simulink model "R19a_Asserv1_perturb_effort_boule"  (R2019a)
settings: Solver=ode15s  StartTime=0.0  StopTime=1  RelTol=1e-3  EnableMultiTasking=on
undefined symbols (not defined in the file): deg, kg, m, manette1_Défaut_sldprt, manette2_Défaut_sldprt, mm, N, rad, s, sigbuilder_block, STL, X, Y, Z
libraries: sm_lib x460, fl_lib x45, nesl_utility x23, simulink x3
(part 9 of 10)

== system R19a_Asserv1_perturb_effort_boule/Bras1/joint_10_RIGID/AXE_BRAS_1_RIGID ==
  ReferenceFrame : sm_lib/Frames and Transforms/Reference Frame
  Solid : sm_lib/Body Elements/Solid  InertiaType=Custom  Mass=0.0015327306958088996  MassUnits=kg  CenterOfMass=[0 0 0]  CenterOfMassUnits=mm  MomentsOfInertia=[0.11359646260705632 0.11359646260705632 0.0017137152305883286]  MomentsOfInertiaUnits=kg*mm^2  ProductsOfInertia=[0 0 0]  ProductsOfInertiaUnits=kg*mm^2  BasedOnType=Density  Density=1000  DensityUnits=kg/(m^3)  DoExposeReferenceFrame=on  SerializedFrames=<Frames/>  GraphicType=FromGeometry  MarkerShape=Sphere  MarkerSize=10  MarkerSizeUnits=m  GraphicVisPropType=SimpleVisualProperties  GraphicDiffuseColor=[0.6470588235294118 0.61960784313725492 0.58823529411764708]  GraphicSpecularColor=[0.5 0.5 0.5 1.0]  GraphicAmbientColor=[0.15 0.15 0.15 1.0]  GraphicEmissiveColor=[0.0 0.0 0.0 1.0]  GraphicShininess=75  GraphicOpacity=1  GeometryShape=FromFile  RectangleSize=[1 1]  RectangleSizeUnits=m  BrickDimensions=[1 1 1]  BrickDimensionUnits=m  CylinderRadius=1  CylinderRadiusUnits=m  CylinderLength=1  CylinderLengthUnits=m  SphereRadius=1  SphereRadiusUnits=m  EllipsoidRadii=[1 1 1]  EllipsoidRadiiUnits=m  ExtrusionCrossSection=[1 1; -1 1; -1 -1; 1 -1]  ExtrusionCrossSectionUnits=m  ExtrusionLength=1  ExtrusionLengthUnits=m  PolygonNumSides=3  PolygonOuterRadius=1  PolygonOuterRadiusUnits=m  ExtGeomFileType=STL  ExtGeomFileName=\STL\AXE BRAS_Défaut_sldprt.STL  ExtGeomFileUnits=mm  RevolutionCrossSection=[1 1; 1 -1; 2 -1; 2 1]  RevolutionCrossSectionUnits=m  RevolutionExtent=Full  RevolutionAngle=180  RevolutionAngleUnits=deg
  F : PMIOPort  Side=Left
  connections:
  Solid/RConn1 -- ReferenceFrame/RConn1 -- F/RConn1

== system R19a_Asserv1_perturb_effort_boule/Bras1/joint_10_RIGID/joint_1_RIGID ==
  ReferenceFrame : sm_lib/Frames and Transforms/Reference Frame
  Solid : sm_lib/Body Elements/Solid  InertiaType=Custom  Mass=0.0062454336323428689  MassUnits=kg  CenterOfMass=[-4.7519597301086606e-06 14.873568128586268 0.2827021501004604]  CenterOfMassUnits=mm  MomentsOfInertia=[0.43544209184236687 0.81590742360241675 0.91424830357082487]  MomentsOfInertiaUnits=kg*mm^2  ProductsOfInertia=[0.0068320776316595647 -4.173068650825101e-06 -7.5142319098046527e-07]  ProductsOfInertiaUnits=kg*mm^2  BasedOnType=Density  Density=1000  DensityUnits=kg/(m^3)  DoExposeReferenceFrame=on  SerializedFrames=<Frames/>  GraphicType=FromGeometry  MarkerShape=Sphere  MarkerSize=10  MarkerSizeUnits=m  GraphicVisPropType=SimpleVisualProperties  GraphicDiffuseColor=[1 1 1]  GraphicSpecularColor=[0.5 0.5 0.5 1.0]  GraphicAmbientColor=[0.15 0.15 0.15 1.0]  GraphicEmissiveColor=[0.0 0.0 0.0 1.0]  GraphicShininess=75  GraphicOpacity=1  GeometryShape=FromFile  RectangleSize=[1 1]  RectangleSizeUnits=m  BrickDimensions=[1 1 1]  BrickDimensionUnits=m  CylinderRadius=1  CylinderRadiusUnits=m  CylinderLength=1  CylinderLengthUnits=m  SphereRadius=1  SphereRadiusUnits=m  EllipsoidRadii=[1 1 1]  EllipsoidRadiiUnits=m  ExtrusionCrossSection=[1 1; -1 1; -1 -1; 1 -1]  ExtrusionCrossSectionUnits=m  ExtrusionLength=1  ExtrusionLengthUnits=m  PolygonNumSides=3  PolygonOuterRadius=1  PolygonOuterRadiusUnits=m  ExtGeomFileType=STL  ExtGeomFileName=\STL\joint_Défaut_sldprt.STL  ExtGeomFileUnits=mm  RevolutionCrossSection=[1 1; 1 -1; 2 -1; 2 1]  RevolutionCrossSectionUnits=m  RevolutionExtent=Full  RevolutionAngle=180  RevolutionAngleUnits=deg
  F : PMIOPort  Side=Left
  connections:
  Solid/RConn1 -- ReferenceFrame/RConn1 -- F/RConn1

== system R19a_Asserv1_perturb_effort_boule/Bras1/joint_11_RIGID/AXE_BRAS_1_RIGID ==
  ReferenceFrame : sm_lib/Frames and Transforms/Reference Frame
  Solid : sm_lib/Body Elements/Solid  InertiaType=Custom  Mass=0.0015327306958088996  MassUnits=kg  CenterOfMass=[0 0 0]  CenterOfMassUnits=mm  MomentsOfInertia=[0.11359646260705632 0.11359646260705632 0.0017137152305883286]  MomentsOfInertiaUnits=kg*mm^2  ProductsOfInertia=[0 0 0]  ProductsOfInertiaUnits=kg*mm^2  BasedOnType=Density  Density=1000  DensityUnits=kg/(m^3)  DoExposeReferenceFrame=on  SerializedFrames=<Frames/>  GraphicType=FromGeometry  MarkerShape=Sphere  MarkerSize=10  MarkerSizeUnits=m  GraphicVisPropType=SimpleVisualProperties  GraphicDiffuseColor=[0.6470588235294118 0.61960784313725492 0.58823529411764708]  GraphicSpecularColor=[0.5 0.5 0.5 1.0]  GraphicAmbientColor=[0.15 0.15 0.15 1.0]  GraphicEmissiveColor=[0.0 0.0 0.0 1.0]  GraphicShininess=75  GraphicOpacity=1  GeometryShape=FromFile  RectangleSize=[1 1]  RectangleSizeUnits=m  BrickDimensions=[1 1 1]  BrickDimensionUnits=m  CylinderRadius=1  CylinderRadiusUnits=m  CylinderLength=1  CylinderLengthUnits=m  SphereRadius=1  SphereRadiusUnits=m  EllipsoidRadii=[1 1 1]  EllipsoidRadiiUnits=m  ExtrusionCrossSection=[1 1; -1 1; -1 -1; 1 -1]  ExtrusionCrossSectionUnits=m  ExtrusionLength=1  ExtrusionLengthUnits=m  PolygonNumSides=3  PolygonOuterRadius=1  PolygonOuterRadiusUnits=m  ExtGeomFileType=STL  ExtGeomFileName=\STL\AXE BRAS_Défaut_sldprt.STL  ExtGeomFileUnits=mm  RevolutionCrossSection=[1 1; 1 -1; 2 -1; 2 1]  RevolutionCrossSectionUnits=m  RevolutionExtent=Full  RevolutionAngle=180  RevolutionAngleUnits=deg
  F : PMIOPort  Side=Left
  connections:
  Solid/RConn1 -- ReferenceFrame/RConn1 -- F/RConn1

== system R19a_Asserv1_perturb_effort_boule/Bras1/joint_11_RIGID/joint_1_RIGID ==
  ReferenceFrame : sm_lib/Frames and Transforms/Reference Frame
  Solid : sm_lib/Body Elements/Solid  InertiaType=Custom  Mass=0.0062454336323428689  MassUnits=kg  CenterOfMass=[-4.7519597301086606e-06 14.873568128586268 0.2827021501004604]  CenterOfMassUnits=mm  MomentsOfInertia=[0.43544209184236687 0.81590742360241675 0.91424830357082487]  MomentsOfInertiaUnits=kg*mm^2  ProductsOfInertia=[0.0068320776316595647 -4.173068650825101e-06 -7.5142319098046527e-07]  ProductsOfInertiaUnits=kg*mm^2  BasedOnType=Density  Density=1000  DensityUnits=kg/(m^3)  DoExposeReferenceFrame=on  SerializedFrames=<Frames/>  GraphicType=FromGeometry  MarkerShape=Sphere  MarkerSize=10  MarkerSizeUnits=m  GraphicVisPropType=SimpleVisualProperties  GraphicDiffuseColor=[1 1 1]  GraphicSpecularColor=[0.5 0.5 0.5 1.0]  GraphicAmbientColor=[0.15 0.15 0.15 1.0]  GraphicEmissiveColor=[0.0 0.0 0.0 1.0]  GraphicShininess=75  GraphicOpacity=1  GeometryShape=FromFile  RectangleSize=[1 1]  RectangleSizeUnits=m  BrickDimensions=[1 1 1]  BrickDimensionUnits=m  CylinderRadius=1  CylinderRadiusUnits=m  CylinderLength=1  CylinderLengthUnits=m  SphereRadius=1  SphereRadiusUnits=m  EllipsoidRadii=[1 1 1]  EllipsoidRadiiUnits=m  ExtrusionCrossSection=[1 1; -1 1; -1 -1; 1 -1]  ExtrusionCrossSectionUnits=m  ExtrusionLength=1  ExtrusionLengthUnits=m  PolygonNumSides=3  PolygonOuterRadius=1  PolygonOuterRadiusUnits=m  ExtGeomFileType=STL  ExtGeomFileName=\STL\joint_Défaut_sldprt.STL  ExtGeomFileUnits=mm  RevolutionCrossSection=[1 1; 1 -1; 2 -1; 2 1]  RevolutionCrossSectionUnits=m  RevolutionExtent=Full  RevolutionAngle=180  RevolutionAngleUnits=deg
  F : PMIOPort  Side=Left
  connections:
  Solid/RConn1 -- ReferenceFrame/RConn1 -- F/RConn1

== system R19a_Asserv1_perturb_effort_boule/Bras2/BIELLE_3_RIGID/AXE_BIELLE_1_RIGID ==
  ReferenceFrame : sm_lib/Frames and Transforms/Reference Frame
  Solid : sm_lib/Body Elements/Solid  InertiaType=Custom  Mass=0.0008880235381781051  MassUnits=kg  CenterOfMass=[0 0 0]  CenterOfMassUnits=mm  MomentsOfInertia=[0.018768660222737772 0.018768660222737772 0.0009874025874388381]  MomentsOfInertiaUnits=kg*mm^2  ProductsOfInertia=[0 0 0]  ProductsOfInertiaUnits=kg*mm^2  BasedOnType=Density  Density=1000  DensityUnits=kg/(m^3)  DoExposeReferenceFrame=on  SerializedFrames=<Frames/>  GraphicType=FromGeometry  MarkerShape=Sphere  MarkerSize=10  MarkerSizeUnits=m  GraphicVisPropType=SimpleVisualProperties  GraphicDiffuseColor=[1 0.94901960784313721 0.90980392156862744]  GraphicSpecularColor=[0.5 0.5 0.5 1.0]  GraphicAmbientColor=[0.15 0.15 0.15 1.0]  GraphicEmissiveColor=[0.0 0.0 0.0 1.0]  GraphicShininess=75  GraphicOpacity=1  GeometryShape=FromFile  RectangleSize=[1 1]  RectangleSizeUnits=m  BrickDimensions=[1 1 1]  BrickDimensionUnits=m  CylinderRadius=1  CylinderRadiusUnits=m  CylinderLength=1  CylinderLengthUnits=m  SphereRadius=1  SphereRadiusUnits=m  EllipsoidRadii=[1 1 1]  EllipsoidRadiiUnits=m  ExtrusionCrossSection=[1 1; -1 1; -1 -1; 1 -1]  ExtrusionCrossSectionUnits=m  ExtrusionLength=1  ExtrusionLengthUnits=m  PolygonNumSides=3  PolygonOuterRadius=1  PolygonOuterRadiusUnits=m  ExtGeomFileType=STL  ExtGeomFileName=\STL\AXE BIELLE_Défaut_sldprt.STL  ExtGeomFileUnits=mm  RevolutionCrossSection=[1 1; 1 -1; 2 -1; 2 1]  RevolutionCrossSectionUnits=m  RevolutionExtent=Full  RevolutionAngle=180  RevolutionAngleUnits=deg
  F : PMIOPort  Side=Left
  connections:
  Solid/RConn1 -- ReferenceFrame/RConn1 -- F/RConn1

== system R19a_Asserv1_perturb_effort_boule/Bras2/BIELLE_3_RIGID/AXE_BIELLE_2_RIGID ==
  ReferenceFrame : sm_lib/Frames and Transforms/Reference Frame
  Solid : sm_lib/Body Elements/Solid  InertiaType=Custom  Mass=0.0008880235381781051  MassUnits=kg  CenterOfMass=[0 0 0]  CenterOfMassUnits=mm  MomentsOfInertia=[0.018768660222737772 0.018768660222737772 0.0009874025874388381]  MomentsOfInertiaUnits=kg*mm^2  ProductsOfInertia=[0 0 0]  ProductsOfInertiaUnits=kg*mm^2  BasedOnType=Density  Density=1000  DensityUnits=kg/(m^3)  DoExposeReferenceFrame=on  SerializedFrames=<Frames/>  GraphicType=FromGeometry  MarkerShape=Sphere  MarkerSize=10  MarkerSizeUnits=m  GraphicVisPropType=SimpleVisualProperties  GraphicDiffuseColor=[1 0.94901960784313721 0.90980392156862744]  GraphicSpecularColor=[0.5 0.5 0.5 1.0]  GraphicAmbientColor=[0.15 0.15 0.15 1.0]  GraphicEmissiveColor=[0.0 0.0 0.0 1.0]  GraphicShininess=75  GraphicOpacity=1  GeometryShape=FromFile  RectangleSize=[1 1]  RectangleSizeUnits=m  BrickDimensions=[1 1 1]  BrickDimensionUnits=m  CylinderRadius=1  CylinderRadiusUnits=m  CylinderLength=1  CylinderLengthUnits=m  SphereRadius=1  SphereRadiusUnits=m  EllipsoidRadii=[1 1 1]  EllipsoidRadiiUnits=m  ExtrusionCrossSection=[1 1; -1 1; -1 -1; 1 -1]  ExtrusionCrossSectionUnits=m  ExtrusionLength=1  ExtrusionLengthUnits=m  PolygonNumSides=3  PolygonOuterRadius=1  PolygonOuterRadiusUnits=m  ExtGeomFileType=STL  ExtGeomFileName=\STL\AXE BIELLE_Défaut_sldprt.STL  ExtGeomFileUnits=mm  RevolutionCrossSection=[1 1; 1 -1; 2 -1; 2 1]  RevolutionCrossSectionUnits=m  RevolutionExtent=Full  RevolutionAngle=180  RevolutionAngleUnits=deg
  F : PMIOPort  Side=Left
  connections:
  Solid/RConn1 -- ReferenceFrame/RConn1 -- F/RConn1

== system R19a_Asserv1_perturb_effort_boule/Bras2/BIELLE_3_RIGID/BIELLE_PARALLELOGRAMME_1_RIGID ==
  ReferenceFrame : sm_lib/Frames and Transforms/Reference Frame
  Solid : sm_lib/Body Elements/Solid  InertiaType=Custom  Mass=0.0079529027635324764  MassUnits=kg  CenterOfMass=[0 3.1653377955585489 0]  CenterOfMassUnits=mm  MomentsOfInertia=[7.7987017961340088 7.8475939194203406 0.14816857834406802]  MomentsOfInertiaUnits=kg*mm^2  ProductsOfInertia=[0 0 0]  ProductsOfInertiaUnits=kg*mm^2  BasedOnType=Density  Density=1000  DensityUnits=kg/(m^3)  DoExposeReferenceFrame=on  SerializedFrames=<Frames/>  GraphicType=FromGeometry  MarkerShape=Sphere  MarkerSize=10  MarkerSizeUnits=m  GraphicVisPropType=SimpleVisualProperties  GraphicDiffuseColor=[0.6 1.0 1.0]  GraphicSpecularColor=[0.5 0.5 0.5 1.0]  GraphicAmbientColor=[0.15 0.15 0.15 1.0]  GraphicEmissiveColor=[0.0 0.0 0.0 1.0]  GraphicShininess=75  GraphicOpacity=1  GeometryShape=FromFile  RectangleSize=[1 1]  RectangleSizeUnits=m  BrickDimensions=[1 1 1]  BrickDimensionUnits=m  CylinderRadius=1  CylinderRadiusUnits=m  CylinderLength=1  CylinderLengthUnits=m  SphereRadius=1  SphereRadiusUnits=m  EllipsoidRadii=[1 1 1]  EllipsoidRadiiUnits=m  ExtrusionCrossSection=[1 1; -1 1; -1 -1; 1 -1]  ExtrusionCrossSectionUnits=m  ExtrusionLength=1  ExtrusionLengthUnits=m  PolygonNumSides=3  PolygonOuterRadius=1  PolygonOuterRadiusUnits=m  ExtGeomFileType=STL  ExtGeomFileName=\STL\BIELLE PARALLELOGRAMME_Défaut_sldprt.STL  ExtGeomFileUnits=mm  RevolutionCrossSection=[1 1; 1 -1; 2 -1; 2 1]  RevolutionCrossSectionUnits=m  RevolutionExtent=Full  RevolutionAngle=180  RevolutionAngleUnits=deg
  F : PMIOPort  Side=Left
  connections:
  Solid/RConn1 -- ReferenceFrame/RConn1 -- F/RConn1

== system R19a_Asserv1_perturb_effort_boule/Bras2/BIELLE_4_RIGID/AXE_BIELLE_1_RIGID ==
  ReferenceFrame : sm_lib/Frames and Transforms/Reference Frame
  Solid : sm_lib/Body Elements/Solid  InertiaType=Custom  Mass=0.0008880235381781051  MassUnits=kg  CenterOfMass=[0 0 0]  CenterOfMassUnits=mm  MomentsOfInertia=[0.018768660222737772 0.018768660222737772 0.0009874025874388381]  MomentsOfInertiaUnits=kg*mm^2  ProductsOfInertia=[0 0 0]  ProductsOfInertiaUnits=kg*mm^2  BasedOnType=Density  Density=1000  DensityUnits=kg/(m^3)  DoExposeReferenceFrame=on  SerializedFrames=<Frames/>  GraphicType=FromGeometry  MarkerShape=Sphere  MarkerSize=10  MarkerSizeUnits=m  GraphicVisPropType=SimpleVisualProperties  GraphicDiffuseColor=[1 0.94901960784313721 0.90980392156862744]  GraphicSpecularColor=[0.5 0.5 0.5 1.0]  GraphicAmbientColor=[0.15 0.15 0.15 1.0]  GraphicEmissiveColor=[0.0 0.0 0.0 1.0]  GraphicShininess=75  GraphicOpacity=1  GeometryShape=FromFile  RectangleSize=[1 1]  RectangleSizeUnits=m  BrickDimensions=[1 1 1]  BrickDimensionUnits=m  CylinderRadius=1  CylinderRadiusUnits=m  CylinderLength=1  CylinderLengthUnits=m  SphereRadius=1  SphereRadiusUnits=m  EllipsoidRadii=[1 1 1]  EllipsoidRadiiUnits=m  ExtrusionCrossSection=[1 1; -1 1; -1 -1; 1 -1]  ExtrusionCrossSectionUnits=m  ExtrusionLength=1  ExtrusionLengthUnits=m  PolygonNumSides=3  PolygonOuterRadius=1  PolygonOuterRadiusUnits=m  ExtGeomFileType=STL  ExtGeomFileName=\STL\AXE BIELLE_Défaut_sldprt.STL  ExtGeomFileUnits=mm  RevolutionCrossSection=[1 1; 1 -1; 2 -1; 2 1]  RevolutionCrossSectionUnits=m  RevolutionExtent=Full  RevolutionAngle=180  RevolutionAngleUnits=deg
  F : PMIOPort  Side=Left
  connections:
  Solid/RConn1 -- ReferenceFrame/RConn1 -- F/RConn1

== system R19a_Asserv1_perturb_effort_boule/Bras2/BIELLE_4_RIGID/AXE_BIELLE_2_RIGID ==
  ReferenceFrame : sm_lib/Frames and Transforms/Reference Frame
  Solid : sm_lib/Body Elements/Solid  InertiaType=Custom  Mass=0.0008880235381781051  MassUnits=kg  CenterOfMass=[0 0 0]  CenterOfMassUnits=mm  MomentsOfInertia=[0.018768660222737772 0.018768660222737772 0.0009874025874388381]  MomentsOfInertiaUnits=kg*mm^2  ProductsOfInertia=[0 0 0]  ProductsOfInertiaUnits=kg*mm^2  BasedOnType=Density  Density=1000  DensityUnits=kg/(m^3)  DoExposeReferenceFrame=on  SerializedFrames=<Frames/>  GraphicType=FromGeometry  MarkerShape=Sphere  MarkerSize=10  MarkerSizeUnits=m  GraphicVisPropType=SimpleVisualProperties  GraphicDiffuseColor=[1 0.94901960784313721 0.90980392156862744]  GraphicSpecularColor=[0.5 0.5 0.5 1.0]  GraphicAmbientColor=[0.15 0.15 0.15 1.0]  GraphicEmissiveColor=[0.0 0.0 0.0 1.0]  GraphicShininess=75  GraphicOpacity=1  GeometryShape=FromFile  RectangleSize=[1 1]  RectangleSizeUnits=m  BrickDimensions=[1 1 1]  BrickDimensionUnits=m  CylinderRadius=1  CylinderRadiusUnits=m  CylinderLength=1  CylinderLengthUnits=m  SphereRadius=1  SphereRadiusUnits=m  EllipsoidRadii=[1 1 1]  EllipsoidRadiiUnits=m  ExtrusionCrossSection=[1 1; -1 1; -1 -1; 1 -1]  ExtrusionCrossSectionUnits=m  ExtrusionLength=1  ExtrusionLengthUnits=m  PolygonNumSides=3  PolygonOuterRadius=1  PolygonOuterRadiusUnits=m  ExtGeomFileType=STL  ExtGeomFileName=\STL\AXE BIELLE_Défaut_sldprt.STL  ExtGeomFileUnits=mm  RevolutionCrossSection=[1 1; 1 -1; 2 -1; 2 1]  RevolutionCrossSectionUnits=m  RevolutionExtent=Full  RevolutionAngle=180  RevolutionAngleUnits=deg
  F : PMIOPort  Side=Left
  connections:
  Solid/RConn1 -- ReferenceFrame/RConn1 -- F/RConn1

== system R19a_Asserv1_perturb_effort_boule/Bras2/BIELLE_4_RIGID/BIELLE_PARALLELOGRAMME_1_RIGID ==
  ReferenceFrame : sm_lib/Frames and Transforms/Reference Frame
  Solid : sm_lib/Body Elements/Solid  InertiaType=Custom  Mass=0.0079529027635324764  MassUnits=kg  CenterOfMass=[0 3.1653377955585489 0]  CenterOfMassUnits=mm  MomentsOfInertia=[7.7987017961340088 7.8475939194203406 0.14816857834406802]  MomentsOfInertiaUnits=kg*mm^2  ProductsOfInertia=[0 0 0]  ProductsOfInertiaUnits=kg*mm^2  BasedOnType=Density  Density=1000  DensityUnits=kg/(m^3)  DoExposeReferenceFrame=on  SerializedFrames=<Frames/>  GraphicType=FromGeometry  MarkerShape=Sphere  MarkerSize=10  MarkerSizeUnits=m  GraphicVisPropType=SimpleVisualProperties  GraphicDiffuseColor=[0.6 1.0 1.0]  GraphicSpecularColor=[0.5 0.5 0.5 1.0]  GraphicAmbientColor=[0.15 0.15 0.15 1.0]  GraphicEmissiveColor=[0.0 0.0 0.0 1.0]  GraphicShininess=75  GraphicOpacity=1  GeometryShape=FromFile  RectangleSize=[1 1]  RectangleSizeUnits=m  BrickDimensions=[1 1 1]  BrickDimensionUnits=m  CylinderRadius=1  CylinderRadiusUnits=m  CylinderLength=1  CylinderLengthUnits=m  SphereRadius=1  SphereRadiusUnits=m  EllipsoidRadii=[1 1 1]  EllipsoidRadiiUnits=m  ExtrusionCrossSection=[1 1; -1 1; -1 -1; 1 -1]  ExtrusionCrossSectionUnits=m  ExtrusionLength=1  ExtrusionLengthUnits=m  PolygonNumSides=3  PolygonOuterRadius=1  PolygonOuterRadiusUnits=m  ExtGeomFileType=STL  ExtGeomFileName=\STL\BIELLE PARALLELOGRAMME_Défaut_sldprt.STL  ExtGeomFileUnits=mm  RevolutionCrossSection=[1 1; 1 -1; 2 -1; 2 1]  RevolutionCrossSectionUnits=m  RevolutionExtent=Full  RevolutionAngle=180  RevolutionAngleUnits=deg
  F : PMIOPort  Side=Left
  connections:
  Solid/RConn1 -- ReferenceFrame/RConn1 -- F/RConn1

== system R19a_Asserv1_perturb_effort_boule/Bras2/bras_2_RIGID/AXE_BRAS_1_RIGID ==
  ReferenceFrame : sm_lib/Frames and Transforms/Reference Frame
  Solid : sm_lib/Body Elements/Solid  InertiaType=Custom  Mass=0.0015327306958088996  MassUnits=kg  CenterOfMass=[0 0 0]  CenterOfMassUnits=mm  MomentsOfInertia=[0.11359646260705632 0.11359646260705632 0.0017137152305883286]  MomentsOfInertiaUnits=kg*mm^2  ProductsOfInertia=[0 0 0]  ProductsOfInertiaUnits=kg*mm^2  BasedOnType=Density  Density=1000  DensityUnits=kg/(m^3)  DoExposeReferenceFrame=on  SerializedFrames=<Frames/>  GraphicType=FromGeometry  MarkerShape=Sphere  MarkerSize=10  MarkerSizeUnits=m  GraphicVisPropType=SimpleVisualProperties  GraphicDiffuseColor=[0.6470588235294118 0.61960784313725492 0.58823529411764708]  GraphicSpecularColor=[0.5 0.5 0.5 1.0]  GraphicAmbientColor=[0.15 0.15 0.15 1.0]  GraphicEmissiveColor=[0.0 0.0 0.0 1.0]  GraphicShininess=75  GraphicOpacity=1  GeometryShape=FromFile  RectangleSize=[1 1]  RectangleSizeUnits=m  BrickDimensions=[1 1 1]  BrickDimensionUnits=m  CylinderRadius=1  CylinderRadiusUnits=m  CylinderLength=1  CylinderLengthUnits=m  SphereRadius=1  SphereRadiusUnits=m  EllipsoidRadii=[1 1 1]  EllipsoidRadiiUnits=m  ExtrusionCrossSection=[1 1; -1 1; -1 -1; 1 -1]  ExtrusionCrossSectionUnits=m  ExtrusionLength=1  ExtrusionLengthUnits=m  PolygonNumSides=3  PolygonOuterRadius=1  PolygonOuterRadiusUnits=m  ExtGeomFileType=STL  ExtGeomFileName=\STL\AXE BRAS_Défaut_sldprt.STL  ExtGeomFileUnits=mm  RevolutionCrossSection=[1 1; 1 -1; 2 -1; 2 1]  RevolutionCrossSectionUnits=m  RevolutionExtent=Full  RevolutionAngle=180  RevolutionAngleUnits=deg
  F : PMIOPort  Side=Left
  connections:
  Solid/RConn1 -- ReferenceFrame/RConn1 -- F/RConn1

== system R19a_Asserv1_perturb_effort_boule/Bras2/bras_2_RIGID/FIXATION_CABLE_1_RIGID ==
  ReferenceFrame : sm_lib/Frames and Transforms/Reference Frame
  Solid : sm_lib/Body Elements/Solid  InertiaType=Custom  Mass=3.2000000000000007e-06  MassUnits=kg  CenterOfMass=[0 0 0.099999999999999992]  CenterOfMassUnits=mm  MomentsOfInertia=[4.2773333333333348e-06 4.2773333333333331e-06 8.5333333333333352e-06]  MomentsOfInertiaUnits=kg*mm^2  ProductsOfInertia=[0 0 0]  ProductsOfInertiaUnits=kg*mm^2  BasedOnType=Density  Density=1000  DensityUnits=kg/(m^3)  DoExposeReferenceFrame=on  SerializedFrames=<Frames/>  GraphicType=FromGeometry  MarkerShape=Sphere  MarkerSize=10  MarkerSizeUnits=m  GraphicVisPropType=SimpleVisualProperties  GraphicDiffuseColor=[0.25098039215686274 0.25098039215686274 0.25098039215686274]  GraphicSpecularColor=[0.5 0.5 0.5 1.0]  GraphicAmbientColor=[0.15 0.15 0.15 1.0]  GraphicEmissiveColor=[0.0 0.0 0.0 1.0]  GraphicShininess=75  GraphicOpacity=1  GeometryShape=FromFile  RectangleSize=[1 1]  RectangleSizeUnits=m  BrickDimensions=[1 1 1]  BrickDimensionUnits=m  CylinderRadius=1  CylinderRadiusUnits=m  CylinderLength=1  CylinderLengthUnits=m  SphereRadius=1  SphereRadiusUnits=m  EllipsoidRadii=[1 1 1]  EllipsoidRadiiUnits=m  ExtrusionCrossSection=[1 1; -1 1; -1 -1; 1 -1]  ExtrusionCrossSectionUnits=m  ExtrusionLength=1  ExtrusionLengthUnits=m  PolygonNumSides=3  PolygonOuterRadius=1  PolygonOuterRadiusUnits=m  ExtGeomFileType=STL  ExtGeomFileName=\STL\FIXATION CABLE_Défaut_sldprt.STL  ExtGeomFileUnits=mm  RevolutionCrossSection=[1 1; 1 -1; 2 -1; 2 1]  RevolutionCrossSectionUnits=m  RevolutionExtent=Full  RevolutionAngle=180  RevolutionAngleUnits=deg
  F : PMIOPort  Side=Left
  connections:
  Solid/RConn1 -- ReferenceFrame/RConn1 -- F/RConn1

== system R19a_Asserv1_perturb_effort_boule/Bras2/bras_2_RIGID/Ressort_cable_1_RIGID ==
  ReferenceFrame : sm_lib/Frames and Transforms/Reference Frame
  Solid : sm_lib/Body Elements/Solid  InertiaType=Custom  Mass=0.0011765814520035881  MassUnits=kg  CenterOfMass=[0.086849073647483815 -0.00090479521327996976 6.9508776157243597]  CenterOfMassUnits=mm  MomentsOfInertia=[0.034952381374405594 0.034338972761516762 0.0097063586011258158]  MomentsOfInertiaUnits=kg*mm^2  ProductsOfInertia=[0.00037229322226744533 1.6947615167207185e-06 2.0937803976811866e-06]  ProductsOfInertiaUnits=kg*mm^2  BasedOnType=Density  Density=1000  DensityUnits=kg/(m^3)  DoExposeReferenceFrame=on  SerializedFrames=<Frames/>  GraphicType=FromGeometry  MarkerShape=Sphere  MarkerSize=10  MarkerSizeUnits=m  GraphicVisPropType=SimpleVisualProperties  GraphicDiffuseColor=[0.6470588235294118 0.61960784313725492 0.58823529411764708]  GraphicSpecularColor=[0.5 0.5 0.5 1.0]  GraphicAmbientColor=[0.15 0.15 0.15 1.0]  GraphicEmissiveColor=[0.0 0.0 0.0 1.0]  GraphicShininess=75  GraphicOpacity=1  GeometryShape=FromFile  RectangleSize=[1 1]  RectangleSizeUnits=m  BrickDimensions=[1 1 1]  BrickDimensionUnits=m  CylinderRadius=1  CylinderRadiusUnits=m  CylinderLength=1  CylinderLengthUnits=m  SphereRadius=1  SphereRadiusUnits=m  EllipsoidRadii=[1 1 1]  EllipsoidRadiiUnits=m  ExtrusionCrossSection=[1 1; -1 1; -1 -1; 1 -1]  ExtrusionCrossSectionUnits=m  ExtrusionLength=1  ExtrusionLengthUnits=m  PolygonNumSides=3  PolygonOuterRadius=1  PolygonOuterRadiusUnits=m  ExtGeomFileType=STL  ExtGeomFileName=\STL\Ressort cable_Défaut_sldprt.STL  ExtGeomFileUnits=mm  RevolutionCrossSection=[1 1; 1 -1; 2 -1; 2 1]  RevolutionCrossSectionUnits=m  RevolutionExtent=Full  RevolutionAngle=180  RevolutionAngleUnits=deg
  F : PMIOPort  Side=Left
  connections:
  Solid/RConn1 -- ReferenceFrame/RConn1 -- F/RConn1

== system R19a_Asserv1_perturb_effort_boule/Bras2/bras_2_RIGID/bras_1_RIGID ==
  ReferenceFrame : sm_lib/Frames and Transforms/Reference Frame
  Solid : sm_lib/Body Elements/Solid  InertiaType=Custom  Mass=0.06566875822643542  MassUnits=kg  CenterOfMass=[23.925748169887701 -4.7774352723885904 0.0071346362933715022]  CenterOfMassUnits=mm  MomentsOfInertia=[75.153076467382206 23.577652078949701 94.231108050856861]  MomentsOfInertiaUnits=kg*mm^2  ProductsOfInertia=[0.01532312637695204 0.0017211125494294708 -5.8798668472039237]  ProductsOfInertiaUnits=kg*mm^2  BasedOnType=Density  Density=1000  DensityUnits=kg/(m^3)  DoExposeReferenceFrame=on  SerializedFrames=<Frames/>  GraphicType=FromGeometry  MarkerShape=Sphere  MarkerSize=10  MarkerSizeUnits=m  GraphicVisPropType=SimpleVisualProperties  GraphicDiffuseColor=[1.0 1.0 0.0]  GraphicSpecularColor=[0.5 0.5 0.5 1.0]  GraphicAmbientColor=[0.15 0.15 0.15 1.0]  GraphicEmissiveColor=[0.0 0.0 0.0 1.0]  GraphicShininess=75  GraphicOpacity=1  GeometryShape=FromFile  RectangleSize=[1 1]  RectangleSizeUnits=m  BrickDimensions=[1 1 1]  BrickDimensionUnits=m  CylinderRadius=1  CylinderRadiusUnits=m  CylinderLength=1  CylinderLengthUnits=m  SphereRadius=1  SphereRadiusUnits=m  EllipsoidRadii=[1 1 1]  EllipsoidRadiiUnits=m  ExtrusionCrossSection=[1 1; -1 1; -1 -1; 1 -1]  ExtrusionCrossSectionUnits=m  ExtrusionLength=1  ExtrusionLengthUnits=m  PolygonNumSides=3  PolygonOuterRadius=1  PolygonOuterRadiusUnits=m  ExtGeomFileType=STL  ExtGeomFileName=\STL\bras_Défaut_sldprt.STL  ExtGeomFileUnits=mm  RevolutionCrossSection=[1 1; 1 -1; 2 -1; 2 1]  RevolutionCrossSectionUnits=m  RevolutionExtent=Full  RevolutionAngle=180  RevolutionAngleUnits=deg
  F : PMIOPort  Side=Left
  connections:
  Solid/RConn1 -- ReferenceFrame/RConn1 -- F/RConn1

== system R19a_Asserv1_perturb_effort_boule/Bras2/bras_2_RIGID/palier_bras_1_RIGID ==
  ReferenceFrame : sm_lib/Frames and Transforms/Reference Frame
  Solid : sm_lib/Body Elements/Solid  InertiaType=Custom  Mass=0.00017920168094851793  MassUnits=kg  CenterOfMass=[-178.32667601154176 39.825618202078154 -20.980989744703667]  CenterOfMassUnits=mm  MomentsOfInertia=[0.0018602253674838991 0.0012789874237151958 0.0012789874237151961]  MomentsOfInertiaUnits=kg*mm^2  ProductsOfInertia=[0 0 0]  ProductsOfInertiaUnits=kg*mm^2  BasedOnType=Density  Density=1000  DensityUnits=kg/(m^3)  DoExposeReferenceFrame=on  SerializedFrames=<Frames/>  GraphicType=FromGeometry  MarkerShape=Sphere  MarkerSize=10  MarkerSizeUnits=m  GraphicVisPropType=SimpleVisualProperties  GraphicDiffuseColor=[1 1 1]  GraphicSpecularColor=[0.5 0.5 0.5 1.0]  GraphicAmbientColor=[0.15 0.15 0.15 1.0]  GraphicEmissiveColor=[0.0 0.0 0.0 1.0]  GraphicShininess=75  GraphicOpacity=1  GeometryShape=FromFile  RectangleSize=[1 1]  RectangleSizeUnits=m  BrickDimensions=[1 1 1]  BrickDimensionUnits=m  CylinderRadius=1  CylinderRadiusUnits=m  CylinderLength=1  CylinderLengthUnits=m  SphereRadius=1  SphereRadiusUnits=m  EllipsoidRadii=[1 1 1]  EllipsoidRadiiUnits=m  ExtrusionCrossSection=[1 1; -1 1; -1 -1; 1 -1]  ExtrusionCrossSectionUnits=m  ExtrusionLength=1  ExtrusionLengthUnits=m  PolygonNumSides=3  PolygonOuterRadius=1  PolygonOuterRadiusUnits=m  ExtGeomFileType=STL  ExtGeomFileName=\STL\palier bras_Défaut_sldprt.STL  ExtGeomFileUnits=mm  RevolutionCrossSection=[1 1; 1 -1; 2 -1; 2 1]  RevolutionCrossSectionUnits=m  RevolutionExtent=Full  RevolutionAngle=180  RevolutionAngleUnits=deg
  F : PMIOPort  Side=Left
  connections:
  Solid/RConn1 -- ReferenceFrame/RConn1 -- F/RConn1

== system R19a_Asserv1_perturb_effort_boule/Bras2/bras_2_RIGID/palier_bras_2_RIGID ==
  ReferenceFrame : sm_lib/Frames and Transforms/Reference Frame
  Solid : sm_lib/Body Elements/Solid  InertiaType=Custom  Mass=0.00017920168094851793  MassUnits=kg  CenterOfMass=[-178.32667601154176 39.825618202078154 -20.980989744703667]  CenterOfMassUnits=mm  MomentsOfInertia=[0.0018602253674838991 0.0012789874237151958 0.0012789874237151961]  MomentsOfInertiaUnits=kg*mm^2  ProductsOfInertia=[0 0 0]  ProductsOfInertiaUnits=kg*mm^2  BasedOnType=Density  Density=1000  DensityUnits=kg/(m^3)  DoExposeReferenceFrame=on  SerializedFrames=<Frames/>  GraphicType=FromGeometry  MarkerShape=Sphere  MarkerSize=10  MarkerSizeUnits=m  GraphicVisPropType=SimpleVisualProperties  GraphicDiffuseColor=[1 1 1]  GraphicSpecularColor=[0.5 0.5 0.5 1.0]  GraphicAmbientColor=[0.15 0.15 0.15 1.0]  GraphicEmissiveColor=[0.0 0.0 0.0 1.0]  GraphicShininess=75  GraphicOpacity=1  GeometryShape=FromFile  RectangleSize=[1 1]  RectangleSizeUnits=m  BrickDimensions=[1 1 1]  BrickDimensionUnits=m  CylinderRadius=1  CylinderRadiusUnits=m  CylinderLength=1  CylinderLengthUnits=m  SphereRadius=1  SphereRadiusUnits=m  EllipsoidRadii=[1 1 1]  EllipsoidRadiiUnits=m  ExtrusionCrossSection=[1 1; -1 1; -1 -1; 1 -1]  ExtrusionCrossSectionUnits=m  ExtrusionLength=1  ExtrusionLengthUnits=m  PolygonNumSides=3  PolygonOuterRadius=1  PolygonOuterRadiusUnits=m  ExtGeomFileType=STL  ExtGeomFileName=\STL\palier bras_Défaut_sldprt.STL  ExtGeomFileUnits=mm  RevolutionCrossSection=[1 1; 1 -1; 2 -1; 2 1]  RevolutionCrossSectionUnits=m  RevolutionExtent=Full  RevolutionAngle=180  RevolutionAngleUnits=deg
  F : PMIOPort  Side=Left
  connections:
  Solid/RConn1 -- ReferenceFrame/RConn1 -- F/RConn1

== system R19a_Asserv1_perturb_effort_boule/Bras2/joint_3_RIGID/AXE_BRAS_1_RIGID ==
  ReferenceFrame : sm_lib/Frames and Transforms/Reference Frame
  Solid : sm_lib/Body Elements/Solid  InertiaType=Custom  Mass=0.0015327306958088996  MassUnits=kg  CenterOfMass=[0 0 0]  CenterOfMassUnits=mm  MomentsOfInertia=[0.11359646260705632 0.11359646260705632 0.0017137152305883286]  MomentsOfInertiaUnits=kg*mm^2  ProductsOfInertia=[0 0 0]  ProductsOfInertiaUnits=kg*mm^2  BasedOnType=Density  Density=1000  DensityUnits=kg/(m^3)  DoExposeReferenceFrame=on  SerializedFrames=<Frames/>  GraphicType=FromGeometry  MarkerShape=Sphere  MarkerSize=10  MarkerSizeUnits=m  GraphicVisPropType=SimpleVisualProperties  GraphicDiffuseColor=[0.6470588235294118 0.61960784313725492 0.58823529411764708]  GraphicSpecularColor=[0.5 0.5 0.5 1.0]  GraphicAmbientColor=[0.15 0.15 0.15 1.0]  GraphicEmissiveColor=[0.0 0.0 0.0 1.0]  GraphicShininess=75  GraphicOpacity=1  GeometryShape=FromFile  RectangleSize=[1 1]  RectangleSizeUnits=m  BrickDimensions=[1 1 1]  BrickDimensionUnits=m  CylinderRadius=1  CylinderRadiusUnits=m  CylinderLength=1  CylinderLengthUnits=m  SphereRadius=1  SphereRadiusUnits=m  EllipsoidRadii=[1 1 1]  EllipsoidRadiiUnits=m  ExtrusionCrossSection=[1 1; -1 1; -1 -1; 1 -1]  ExtrusionCrossSectionUnits=m  ExtrusionLength=1  ExtrusionLengthUnits=m  PolygonNumSides=3  PolygonOuterRadius=1  PolygonOuterRadiusUnits=m  ExtGeomFileType=STL  ExtGeomFileName=\STL\AXE BRAS_Défaut_sldprt.STL  ExtGeomFileUnits=mm  RevolutionCrossSection=[1 1; 1 -1; 2 -1; 2 1]  RevolutionCrossSectionUnits=m  RevolutionExtent=Full  RevolutionAngle=180  RevolutionAngleUnits=deg
  F : PMIOPort  Side=Left
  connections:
  Solid/RConn1 -- ReferenceFrame/RConn1 -- F/RConn1

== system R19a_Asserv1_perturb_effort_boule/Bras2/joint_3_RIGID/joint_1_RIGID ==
  ReferenceFrame : sm_lib/Frames and Transforms/Reference Frame
  Solid : sm_lib/Body Elements/Solid  InertiaType=Custom  Mass=0.0062454336323428689  MassUnits=kg  CenterOfMass=[-4.7519597301086606e-06 14.873568128586268 0.2827021501004604]  CenterOfMassUnits=mm  MomentsOfInertia=[0.43544209184236687 0.81590742360241675 0.91424830357082487]  MomentsOfInertiaUnits=kg*mm^2  ProductsOfInertia=[0.0068320776316595647 -4.173068650825101e-06 -7.5142319098046527e-07]  ProductsOfInertiaUnits=kg*mm^2  BasedOnType=Density  Density=1000  DensityUnits=kg/(m^3)  DoExposeReferenceFrame=on  SerializedFrames=<Frames/>  GraphicType=FromGeometry  MarkerShape=Sphere  MarkerSize=10  MarkerSizeUnits=m  GraphicVisPropType=SimpleVisualProperties  GraphicDiffuseColor=[1 1 1]  GraphicSpecularColor=[0.5 0.5 0.5 1.0]  GraphicAmbientColor=[0.15 0.15 0.15 1.0]  GraphicEmissiveColor=[0.0 0.0 0.0 1.0]  GraphicShininess=75  GraphicOpacity=1  GeometryShape=FromFile  RectangleSize=[1 1]  RectangleSizeUnits=m  BrickDimensions=[1 1 1]  BrickDimensionUnits=m  CylinderRadius=1  CylinderRadiusUnits=m  CylinderLength=1  CylinderLengthUnits=m  SphereRadius=1  SphereRadiusUnits=m  EllipsoidRadii=[1 1 1]  EllipsoidRadiiUnits=m  ExtrusionCrossSection=[1 1; -1 1; -1 -1; 1 -1]  ExtrusionCrossSectionUnits=m  ExtrusionLength=1  ExtrusionLengthUnits=m  PolygonNumSides=3  PolygonOuterRadius=1  PolygonOuterRadiusUnits=m  ExtGeomFileType=STL  ExtGeomFileName=\STL\joint_Défaut_sldprt.STL  ExtGeomFileUnits=mm  RevolutionCrossSection=[1 1; 1 -1; 2 -1; 2 1]  RevolutionCrossSectionUnits=m  RevolutionExtent=Full  RevolutionAngle=180  RevolutionAngleUnits=deg
  F : PMIOPort  Side=Left
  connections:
  Solid/RConn1 -- ReferenceFrame/RConn1 -- F/RConn1

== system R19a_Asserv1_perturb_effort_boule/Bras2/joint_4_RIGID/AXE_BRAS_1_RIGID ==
  ReferenceFrame : sm_lib/Frames and Transforms/Reference Frame
  Solid : sm_lib/Body Elements/Solid  InertiaType=Custom  Mass=0.0015327306958088996  MassUnits=kg  CenterOfMass=[0 0 0]  CenterOfMassUnits=mm  MomentsOfInertia=[0.11359646260705632 0.11359646260705632 0.0017137152305883286]  MomentsOfInertiaUnits=kg*mm^2  ProductsOfInertia=[0 0 0]  ProductsOfInertiaUnits=kg*mm^2  BasedOnType=Density  Density=1000  DensityUnits=kg/(m^3)  DoExposeReferenceFrame=on  SerializedFrames=<Frames/>  GraphicType=FromGeometry  MarkerShape=Sphere  MarkerSize=10  MarkerSizeUnits=m  GraphicVisPropType=SimpleVisualProperties  GraphicDiffuseColor=[0.6470588235294118 0.61960784313725492 0.58823529411764708]  GraphicSpecularColor=[0.5 0.5 0.5 1.0]  GraphicAmbientColor=[0.15 0.15 0.15 1.0]  GraphicEmissiveColor=[0.0 0.0 0.0 1.0]  GraphicShininess=75  GraphicOpacity=1  GeometryShape=FromFile  RectangleSize=[1 1]  RectangleSizeUnits=m  BrickDimensions=[1 1 1]  BrickDimensionUnits=m  CylinderRadius=1  CylinderRadiusUnits=m  CylinderLength=1  CylinderLengthUnits=m  SphereRadius=1  SphereRadiusUnits=m  EllipsoidRadii=[1 1 1]  EllipsoidRadiiUnits=m  ExtrusionCrossSection=[1 1; -1 1; -1 -1; 1 -1]  ExtrusionCrossSectionUnits=m  ExtrusionLength=1  ExtrusionLengthUnits=m  PolygonNumSides=3  PolygonOuterRadius=1  PolygonOuterRadiusUnits=m  ExtGeomFileType=STL  ExtGeomFileName=\STL\AXE BRAS_Défaut_sldprt.STL  ExtGeomFileUnits=mm  RevolutionCrossSection=[1 1; 1 -1; 2 -1; 2 1]  RevolutionCrossSectionUnits=m  RevolutionExtent=Full  RevolutionAngle=180  RevolutionAngleUnits=deg
  F : PMIOPort  Side=Left
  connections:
  Solid/RConn1 -- ReferenceFrame/RConn1 -- F/RConn1

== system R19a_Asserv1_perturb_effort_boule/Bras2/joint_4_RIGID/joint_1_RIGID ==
  ReferenceFrame : sm_lib/Frames and Transforms/Reference Frame
  Solid : sm_lib/Body Elements/Solid  InertiaType=Custom  Mass=0.0062454336323428689  MassUnits=kg  CenterOfMass=[-4.7519597301086606e-06 14.873568128586268 0.2827021501004604]  CenterOfMassUnits=mm  MomentsOfInertia=[0.43544209184236687 0.81590742360241675 0.91424830357082487]  MomentsOfInertiaUnits=kg*mm^2  ProductsOfInertia=[0.0068320776316595647 -4.173068650825101e-06 -7.5142319098046527e-07]  ProductsOfInertiaUnits=kg*mm^2  BasedOnType=Density  Density=1000  DensityUnits=kg/(m^3)  DoExposeReferenceFrame=on  SerializedFrames=<Frames/>  GraphicType=FromGeometry  MarkerShape=Sphere  MarkerSize=10  MarkerSizeUnits=m  GraphicVisPropType=SimpleVisualProperties  GraphicDiffuseColor=[1 1 1]  GraphicSpecularColor=[0.5 0.5 0.5 1.0]  GraphicAmbientColor=[0.15 0.15 0.15 1.0]  GraphicEmissiveColor=[0.0 0.0 0.0 1.0]  GraphicShininess=75  GraphicOpacity=1  GeometryShape=FromFile  RectangleSize=[1 1]  RectangleSizeUnits=m  BrickDimensions=[1 1 1]  BrickDimensionUnits=m  CylinderRadius=1  CylinderRadiusUnits=m  CylinderLength=1  CylinderLengthUnits=m  SphereRadius=1  SphereRadiusUnits=m  EllipsoidRadii=[1 1 1]  EllipsoidRadiiUnits=m  ExtrusionCrossSection=[1 1; -1 1; -1 -1; 1 -1]  ExtrusionCrossSectionUnits=m  ExtrusionLength=1  ExtrusionLengthUnits=m  PolygonNumSides=3  PolygonOuterRadius=1  PolygonOuterRadiusUnits=m  ExtGeomFileType=STL  ExtGeomFileName=\STL\joint_Défaut_sldprt.STL  ExtGeomFileUnits=mm  RevolutionCrossSection=[1 1; 1 -1; 2 -1; 2 1]  RevolutionCrossSectionUnits=m  RevolutionExtent=Full  RevolutionAngle=180  RevolutionAngleUnits=deg
  F : PMIOPort  Side=Left
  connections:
  Solid/RConn1 -- ReferenceFrame/RConn1 -- F/RConn1

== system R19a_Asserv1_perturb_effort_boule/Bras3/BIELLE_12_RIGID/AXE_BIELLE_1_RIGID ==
  ReferenceFrame : sm_lib/Frames and Transforms/Reference Frame
  Solid : sm_lib/Body Elements/Solid  InertiaType=Custom  Mass=0.0008880235381781051  MassUnits=kg  CenterOfMass=[0 0 0]  CenterOfMassUnits=mm  MomentsOfInertia=[0.018768660222737772 0.018768660222737772 0.0009874025874388381]  MomentsOfInertiaUnits=kg*mm^2  ProductsOfInertia=[0 0 0]  ProductsOfInertiaUnits=kg*mm^2  BasedOnType=Density  Density=1000  DensityUnits=kg/(m^3)  DoExposeReferenceFrame=on  SerializedFrames=<Frames/>  GraphicType=FromGeometry  MarkerShape=Sphere  MarkerSize=10  MarkerSizeUnits=m  GraphicVisPropType=SimpleVisualProperties  GraphicDiffuseColor=[1 0.94901960784313721 0.90980392156862744]  GraphicSpecularColor=[0.5 0.5 0.5 1.0]  GraphicAmbientColor=[0.15 0.15 0.15 1.0]  GraphicEmissiveColor=[0.0 0.0 0.0 1.0]  GraphicShininess=75  GraphicOpacity=1  GeometryShape=FromFile  RectangleSize=[1 1]  RectangleSizeUnits=m  BrickDimensions=[1 1 1]  BrickDimensionUnits=m  CylinderRadius=1  CylinderRadiusUnits=m  CylinderLength=1  CylinderLengthUnits=m  SphereRadius=1  SphereRadiusUnits=m  EllipsoidRadii=[1 1 1]  EllipsoidRadiiUnits=m  ExtrusionCrossSection=[1 1; -1 1; -1 -1; 1 -1]  ExtrusionCrossSectionUnits=m  ExtrusionLength=1  ExtrusionLengthUnits=m  PolygonNumSides=3  PolygonOuterRadius=1  PolygonOuterRadiusUnits=m  ExtGeomFileType=STL  ExtGeomFileName=\STL\AXE BIELLE_Défaut_sldprt.STL  ExtGeomFileUnits=mm  RevolutionCrossSection=[1 1; 1 -1; 2 -1; 2 1]  RevolutionCrossSectionUnits=m  RevolutionExtent=Full  RevolutionAngle=180  RevolutionAngleUnits=deg
  F : PMIOPort  Side=Left
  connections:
  Solid/RConn1 -- ReferenceFrame/RConn1 -- F/RConn1

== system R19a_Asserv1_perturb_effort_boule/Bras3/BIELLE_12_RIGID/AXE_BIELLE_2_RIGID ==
  ReferenceFrame : sm_lib/Frames and Transforms/Reference Frame
  Solid : sm_lib/Body Elements/Solid  InertiaType=Custom  Mass=0.0008880235381781051  MassUnits=kg  CenterOfMass=[0 0 0]  CenterOfMassUnits=mm  MomentsOfInertia=[0.018768660222737772 0.018768660222737772 0.0009874025874388381]  MomentsOfInertiaUnits=kg*mm^2  ProductsOfInertia=[0 0 0]  ProductsOfInertiaUnits=kg*mm^2  BasedOnType=Density  Density=1000  DensityUnits=kg/(m^3)  DoExposeReferenceFrame=on  SerializedFrames=<Frames/>  GraphicType=FromGeometry  MarkerShape=Sphere  MarkerSize=10  MarkerSizeUnits=m  GraphicVisPropType=SimpleVisualProperties  GraphicDiffuseColor=[1 0.94901960784313721 0.90980392156862744]  GraphicSpecularColor=[0.5 0.5 0.5 1.0]  GraphicAmbientColor=[0.15 0.15 0.15 1.0]  GraphicEmissiveColor=[0.0 0.0 0.0 1.0]  GraphicShininess=75  GraphicOpacity=1  GeometryShape=FromFile  RectangleSize=[1 1]  RectangleSizeUnits=m  BrickDimensions=[1 1 1]  BrickDimensionUnits=m  CylinderRadius=1  CylinderRadiusUnits=m  CylinderLength=1  CylinderLengthUnits=m  SphereRadius=1  SphereRadiusUnits=m  EllipsoidRadii=[1 1 1]  EllipsoidRadiiUnits=m  ExtrusionCrossSection=[1 1; -1 1; -1 -1; 1 -1]  ExtrusionCrossSectionUnits=m  ExtrusionLength=1  ExtrusionLengthUnits=m  PolygonNumSides=3  PolygonOuterRadius=1  PolygonOuterRadiusUnits=m  ExtGeomFileType=STL  ExtGeomFileName=\STL\AXE BIELLE_Défaut_sldprt.STL  ExtGeomFileUnits=mm  RevolutionCrossSection=[1 1; 1 -1; 2 -1; 2 1]  RevolutionCrossSectionUnits=m  RevolutionExtent=Full  RevolutionAngle=180  RevolutionAngleUnits=deg
  F : PMIOPort  Side=Left
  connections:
  Solid/RConn1 -- ReferenceFrame/RConn1 -- F/RConn1

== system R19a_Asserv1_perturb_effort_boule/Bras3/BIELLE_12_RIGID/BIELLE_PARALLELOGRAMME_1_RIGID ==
  ReferenceFrame : sm_lib/Frames and Transforms/Reference Frame
  Solid : sm_lib/Body Elements/Solid  InertiaType=Custom  Mass=0.0079529027635324764  MassUnits=kg  CenterOfMass=[0 3.1653377955585489 0]  CenterOfMassUnits=mm  MomentsOfInertia=[7.7987017961340088 7.8475939194203406 0.14816857834406802]  MomentsOfInertiaUnits=kg*mm^2  ProductsOfInertia=[0 0 0]  ProductsOfInertiaUnits=kg*mm^2  BasedOnType=Density  Density=1000  DensityUnits=kg/(m^3)  DoExposeReferenceFrame=on  SerializedFrames=<Frames/>  GraphicType=FromGeometry  MarkerShape=Sphere  MarkerSize=10  MarkerSizeUnits=m  GraphicVisPropType=SimpleVisualProperties  GraphicDiffuseColor=[0.6 1.0 1.0]  GraphicSpecularColor=[0.5 0.5 0.5 1.0]  GraphicAmbientColor=[0.15 0.15 0.15 1.0]  GraphicEmissiveColor=[0.0 0.0 0.0 1.0]  GraphicShininess=75  GraphicOpacity=1  GeometryShape=FromFile  RectangleSize=[1 1]  RectangleSizeUnits=m  BrickDimensions=[1 1 1]  BrickDimensionUnits=m  CylinderRadius=1  CylinderRadiusUnits=m  CylinderLength=1  CylinderLengthUnits=m  SphereRadius=1  SphereRadiusUnits=m  EllipsoidRadii=[1 1 1]  EllipsoidRadiiUnits=m  ExtrusionCrossSection=[1 1; -1 1; -1 -1; 1 -1]  ExtrusionCrossSectionUnits=m  ExtrusionLength=1  ExtrusionLengthUnits=m  PolygonNumSides=3  PolygonOuterRadius=1  PolygonOuterRadiusUnits=m  ExtGeomFileType=STL  ExtGeomFileName=\STL\BIELLE PARALLELOGRAMME_Défaut_sldprt.STL  ExtGeomFileUnits=mm  RevolutionCrossSection=[1 1; 1 -1; 2 -1; 2 1]  RevolutionCrossSectionUnits=m  RevolutionExtent=Full  RevolutionAngle=180  RevolutionAngleUnits=deg
  F : PMIOPort  Side=Left
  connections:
  Solid/RConn1 -- ReferenceFrame/RConn1 -- F/RConn1

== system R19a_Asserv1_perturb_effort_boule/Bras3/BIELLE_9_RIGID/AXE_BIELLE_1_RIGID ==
  ReferenceFrame : sm_lib/Frames and Transforms/Reference Frame
  Solid : sm_lib/Body Elements/Solid  InertiaType=Custom  Mass=0.0008880235381781051  MassUnits=kg  CenterOfMass=[0 0 0]  CenterOfMassUnits=mm  MomentsOfInertia=[0.018768660222737772 0.018768660222737772 0.0009874025874388381]  MomentsOfInertiaUnits=kg*mm^2  ProductsOfInertia=[0 0 0]  ProductsOfInertiaUnits=kg*mm^2  BasedOnType=Density  Density=1000  DensityUnits=kg/(m^3)  DoExposeReferenceFrame=on  SerializedFrames=<Frames/>  GraphicType=FromGeometry  MarkerShape=Sphere  MarkerSize=10  MarkerSizeUnits=m  GraphicVisPropType=SimpleVisualProperties  GraphicDiffuseColor=[1 0.94901960784313721 0.90980392156862744]  GraphicSpecularColor=[0.5 0.5 0.5 1.0]  GraphicAmbientColor=[0.15 0.15 0.15 1.0]  GraphicEmissiveColor=[0.0 0.0 0.0 1.0]  GraphicShininess=75  GraphicOpacity=1  GeometryShape=FromFile  RectangleSize=[1 1]  RectangleSizeUnits=m  BrickDimensions=[1 1 1]  BrickDimensionUnits=m  CylinderRadius=1  CylinderRadiusUnits=m  CylinderLength=1  CylinderLengthUnits=m  SphereRadius=1  SphereRadiusUnits=m  EllipsoidRadii=[1 1 1]  EllipsoidRadiiUnits=m  ExtrusionCrossSection=[1 1; -1 1; -1 -1; 1 -1]  ExtrusionCrossSectionUnits=m  ExtrusionLength=1  ExtrusionLengthUnits=m  PolygonNumSides=3  PolygonOuterRadius=1  PolygonOuterRadiusUnits=m  ExtGeomFileType=STL  ExtGeomFileName=\STL\AXE BIELLE_Défaut_sldprt.STL  ExtGeomFileUnits=mm  RevolutionCrossSection=[1 1; 1 -1; 2 -1; 2 1]  RevolutionCrossSectionUnits=m  RevolutionExtent=Full  RevolutionAngle=180  RevolutionAngleUnits=deg
  F : PMIOPort  Side=Left
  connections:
  Solid/RConn1 -- ReferenceFrame/RConn1 -- F/RConn1

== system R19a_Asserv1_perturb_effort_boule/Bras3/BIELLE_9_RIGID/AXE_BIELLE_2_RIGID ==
  ReferenceFrame : sm_lib/Frames and Transforms/Reference Frame
  Solid : sm_lib/Body Elements/Solid  InertiaType=Custom  Mass=0.0008880235381781051  MassUnits=kg  CenterOfMass=[0 0 0]  CenterOfMassUnits=mm  MomentsOfInertia=[0.018768660222737772 0.018768660222737772 0.0009874025874388381]  MomentsOfInertiaUnits=kg*mm^2  ProductsOfInertia=[0 0 0]  ProductsOfInertiaUnits=kg*mm^2  BasedOnType=Density  Density=1000  DensityUnits=kg/(m^3)  DoExposeReferenceFrame=on  SerializedFrames=<Frames/>  GraphicType=FromGeometry  MarkerShape=Sphere  MarkerSize=10  MarkerSizeUnits=m  GraphicVisPropType=SimpleVisualProperties  GraphicDiffuseColor=[1 0.94901960784313721 0.90980392156862744]  GraphicSpecularColor=[0.5 0.5 0.5 1.0]  GraphicAmbientColor=[0.15 0.15 0.15 1.0]  GraphicEmissiveColor=[0.0 0.0 0.0 1.0]  GraphicShininess=75  GraphicOpacity=1  GeometryShape=FromFile  RectangleSize=[1 1]  RectangleSizeUnits=m  BrickDimensions=[1 1 1]  BrickDimensionUnits=m  CylinderRadius=1  CylinderRadiusUnits=m  CylinderLength=1  CylinderLengthUnits=m  SphereRadius=1  SphereRadiusUnits=m  EllipsoidRadii=[1 1 1]  EllipsoidRadiiUnits=m  ExtrusionCrossSection=[1 1; -1 1; -1 -1; 1 -1]  ExtrusionCrossSectionUnits=m  ExtrusionLength=1  ExtrusionLengthUnits=m  PolygonNumSides=3  PolygonOuterRadius=1  PolygonOuterRadiusUnits=m  ExtGeomFileType=STL  ExtGeomFileName=\STL\AXE BIELLE_Défaut_sldprt.STL  ExtGeomFileUnits=mm  RevolutionCrossSection=[1 1; 1 -1; 2 -1; 2 1]  RevolutionCrossSectionUnits=m  RevolutionExtent=Full  RevolutionAngle=180  RevolutionAngleUnits=deg
  F : PMIOPort  Side=Left
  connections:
  Solid/RConn1 -- ReferenceFrame/RConn1 -- F/RConn1

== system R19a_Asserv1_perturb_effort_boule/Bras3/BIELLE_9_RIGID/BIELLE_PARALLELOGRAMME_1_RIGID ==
  ReferenceFrame : sm_lib/Frames and Transforms/Reference Frame
  Solid : sm_lib/Body Elements/Solid  InertiaType=Custom  Mass=0.0079529027635324764  MassUnits=kg  CenterOfMass=[0 3.1653377955585489 0]  CenterOfMassUnits=mm  MomentsOfInertia=[7.7987017961340088 7.8475939194203406 0.14816857834406802]  MomentsOfInertiaUnits=kg*mm^2  ProductsOfInertia=[0 0 0]  ProductsOfInertiaUnits=kg*mm^2  BasedOnType=Density  Density=1000  DensityUnits=kg/(m^3)  DoExposeReferenceFrame=on  SerializedFrames=<Frames/>  GraphicType=FromGeometry  MarkerShape=Sphere  MarkerSize=10  MarkerSizeUnits=m  GraphicVisPropType=SimpleVisualProperties  GraphicDiffuseColor=[0.6 1.0 1.0]  GraphicSpecularColor=[0.5 0.5 0.5 1.0]  GraphicAmbientColor=[0.15 0.15 0.15 1.0]  GraphicEmissiveColor=[0.0 0.0 0.0 1.0]  GraphicShininess=75  GraphicOpacity=1  GeometryShape=FromFile  RectangleSize=[1 1]  RectangleSizeUnits=m  BrickDimensions=[1 1 1]  BrickDimensionUnits=m  CylinderRadius=1  CylinderRadiusUnits=m  CylinderLength=1  CylinderLengthUnits=m  SphereRadius=1  SphereRadiusUnits=m  EllipsoidRadii=[1 1 1]  EllipsoidRadiiUnits=m  ExtrusionCrossSection=[1 1; -1 1; -1 -1; 1 -1]  ExtrusionCrossSectionUnits=m  ExtrusionLength=1  ExtrusionLengthUnits=m  PolygonNumSides=3  PolygonOuterRadius=1  PolygonOuterRadiusUnits=m  ExtGeomFileType=STL  ExtGeomFileName=\STL\BIELLE PARALLELOGRAMME_Défaut_sldprt.STL  ExtGeomFileUnits=mm  RevolutionCrossSection=[1 1; 1 -1; 2 -1; 2 1]  RevolutionCrossSectionUnits=m  RevolutionExtent=Full  RevolutionAngle=180  RevolutionAngleUnits=deg
  F : PMIOPort  Side=Left
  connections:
  Solid/RConn1 -- ReferenceFrame/RConn1 -- F/RConn1

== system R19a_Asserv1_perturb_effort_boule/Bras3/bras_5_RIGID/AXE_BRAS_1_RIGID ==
  ReferenceFrame : sm_lib/Frames and Transforms/Reference Frame
  Solid : sm_lib/Body Elements/Solid  InertiaType=Custom  Mass=0.0015327306958088996  MassUnits=kg  CenterOfMass=[0 0 0]  CenterOfMassUnits=mm  MomentsOfInertia=[0.11359646260705632 0.11359646260705632 0.0017137152305883286]  MomentsOfInertiaUnits=kg*mm^2  ProductsOfInertia=[0 0 0]  ProductsOfInertiaUnits=kg*mm^2  BasedOnType=Density  Density=1000  DensityUnits=kg/(m^3)  DoExposeReferenceFrame=on  SerializedFrames=<Frames/>  GraphicType=FromGeometry  MarkerShape=Sphere  MarkerSize=10  MarkerSizeUnits=m  GraphicVisPropType=SimpleVisualProperties  GraphicDiffuseColor=[0.6470588235294118 0.61960784313725492 0.58823529411764708]  GraphicSpecularColor=[0.5 0.5 0.5 1.0]  GraphicAmbientColor=[0.15 0.15 0.15 1.0]  GraphicEmissiveColor=[0.0 0.0 0.0 1.0]  GraphicShininess=75  GraphicOpacity=1  GeometryShape=FromFile  RectangleSize=[1 1]  RectangleSizeUnits=m  BrickDimensions=[1 1 1]  BrickDimensionUnits=m  CylinderRadius=1  CylinderRadiusUnits=m  CylinderLength=1  CylinderLengthUnits=m  SphereRadius=1  SphereRadiusUnits=m  EllipsoidRadii=[1 1 1]  EllipsoidRadiiUnits=m  ExtrusionCrossSection=[1 1; -1 1; -1 -1; 1 -1]  ExtrusionCrossSectionUnits=m  ExtrusionLength=1  ExtrusionLengthUnits=m  PolygonNumSides=3  PolygonOuterRadius=1  PolygonOuterRadiusUnits=m  ExtGeomFileType=STL  ExtGeomFileName=\STL\AXE BRAS_Défaut_sldprt.STL  ExtGeomFileUnits=mm  RevolutionCrossSection=[1 1; 1 -1; 2 -1; 2 1]  RevolutionCrossSectionUnits=m  RevolutionExtent=Full  RevolutionAngle=180  RevolutionAngleUnits=deg
  F : PMIOPort  Side=Left
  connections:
  Solid/RConn1 -- ReferenceFrame/RConn1 -- F/RConn1

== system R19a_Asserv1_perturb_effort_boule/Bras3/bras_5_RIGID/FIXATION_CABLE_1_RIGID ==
  ReferenceFrame : sm_lib/Frames and Transforms/Reference Frame
  Solid : sm_lib/Body Elements/Solid  InertiaType=Custom  Mass=3.2000000000000007e-06  MassUnits=kg  CenterOfMass=[0 0 0.099999999999999992]  CenterOfMassUnits=mm  MomentsOfInertia=[4.2773333333333348e-06 4.2773333333333331e-06 8.5333333333333352e-06]  MomentsOfInertiaUnits=kg*mm^2  ProductsOfInertia=[0 0 0]  ProductsOfInertiaUnits=kg*mm^2  BasedOnType=Density  Density=1000  DensityUnits=kg/(m^3)  DoExposeReferenceFrame=on  SerializedFrames=<Frames/>  GraphicType=FromGeometry  MarkerShape=Sphere  MarkerSize=10  MarkerSizeUnits=m  GraphicVisPropType=SimpleVisualProperties  GraphicDiffuseColor=[0.25098039215686274 0.25098039215686274 0.25098039215686274]  GraphicSpecularColor=[0.5 0.5 0.5 1.0]  GraphicAmbientColor=[0.15 0.15 0.15 1.0]  GraphicEmissiveColor=[0.0 0.0 0.0 1.0]  GraphicShininess=75  GraphicOpacity=1  GeometryShape=FromFile  RectangleSize=[1 1]  RectangleSizeUnits=m  BrickDimensions=[1 1 1]  BrickDimensionUnits=m  CylinderRadius=1  CylinderRadiusUnits=m  CylinderLength=1  CylinderLengthUnits=m  SphereRadius=1  SphereRadiusUnits=m  EllipsoidRadii=[1 1 1]  EllipsoidRadiiUnits=m  ExtrusionCrossSection=[1 1; -1 1; -1 -1; 1 -1]  ExtrusionCrossSectionUnits=m  ExtrusionLength=1  ExtrusionLengthUnits=m  PolygonNumSides=3  PolygonOuterRadius=1  PolygonOuterRadiusUnits=m  ExtGeomFileType=STL  ExtGeomFileName=\STL\FIXATION CABLE_Défaut_sldprt.STL  ExtGeomFileUnits=mm  RevolutionCrossSection=[1 1; 1 -1; 2 -1; 2 1]  RevolutionCrossSectionUnits=m  RevolutionExtent=Full  RevolutionAngle=180  RevolutionAngleUnits=deg
  F : PMIOPort  Side=Left
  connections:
  Solid/RConn1 -- ReferenceFrame/RConn1 -- F/RConn1
